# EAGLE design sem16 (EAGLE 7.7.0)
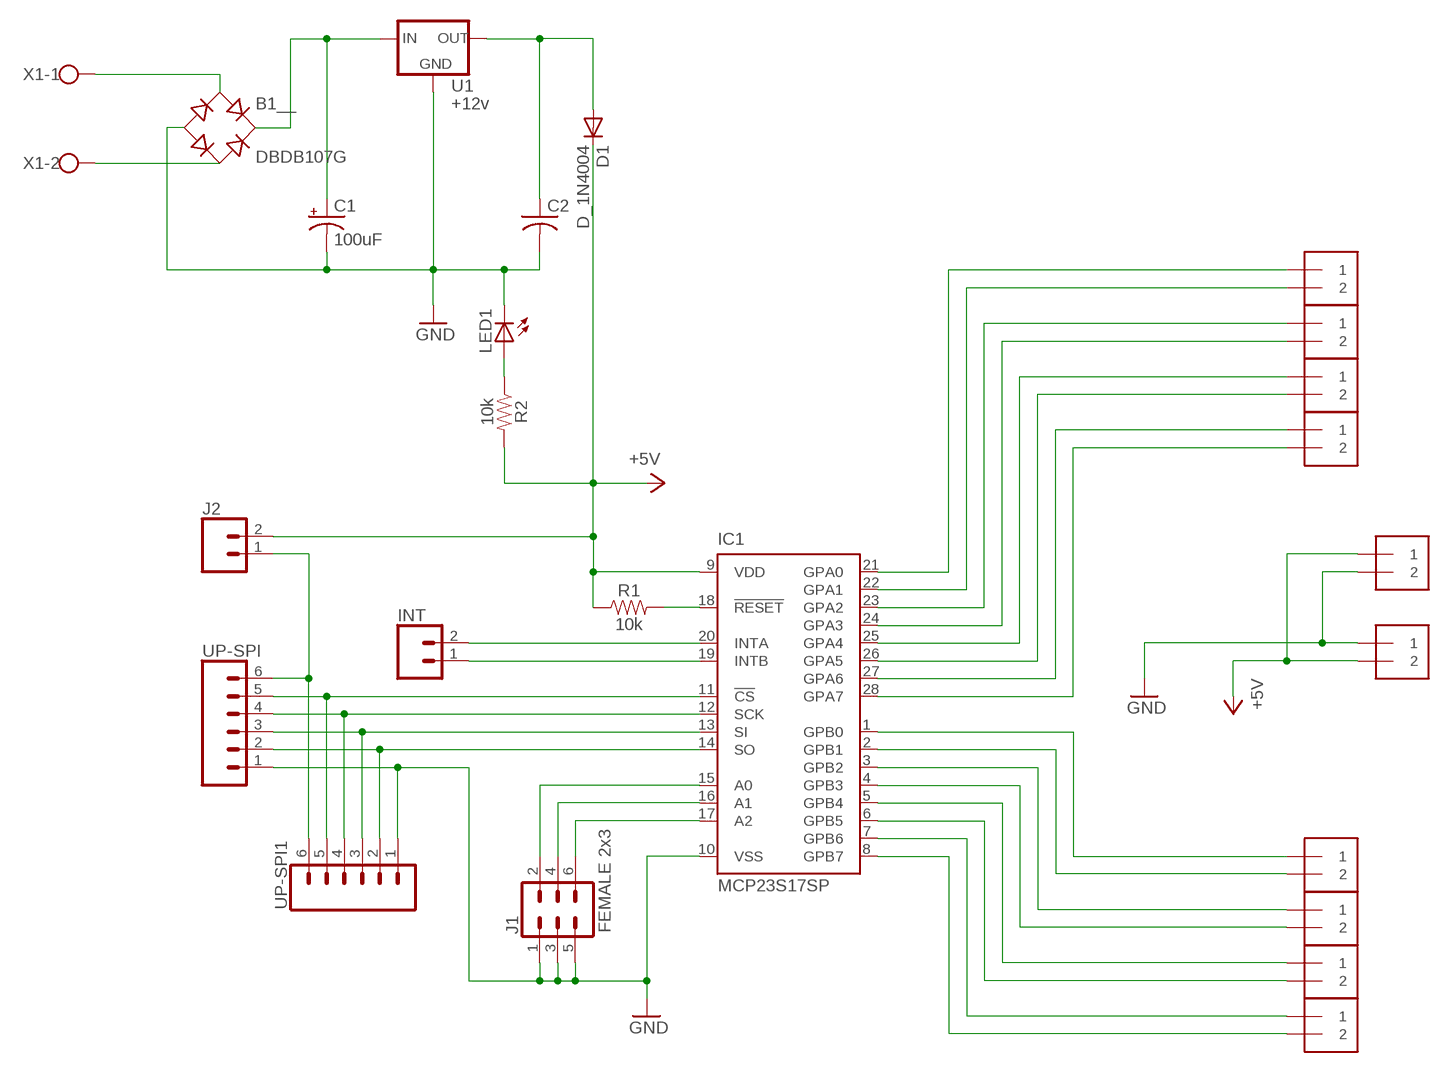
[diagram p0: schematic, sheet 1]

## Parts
+5V  1X2-3.5MM  [1X2-3.5MM]
A0_A1  1X2-3.5MM  [1X2-3.5MM]
A2_A3  1X2-3.5MM  [1X2-3.5MM]
A4_A5  1X2-3.5MM  [1X2-3.5MM]
A6_A7  1X2-3.5MM  [1X2-3.5MM]
B0_B1  1X2-3.5MM  [1X2-3.5MM]
B1__  DBDB107G  [DB]
B2_B3  1X2-3.5MM  [1X2-3.5MM]
B4_B5  1X2-3.5MM  [1X2-3.5MM]
B6_B7  1X2-3.5MM  [1X2-3.5MM]
C1  100uF  100UF-POLAR-RADIAL-2.5MM-25V-20%  [CPOL-RADIAL-2.5MM-6.5MM]
C2  C-US025-025X050  [C025-025X050]
D1  D_1N4004  [DO41-10]
GND  1X2-3.5MM  [1X2-3.5MM]
IC1  MCP23S17SP  [DIL28-3]
INT  CONN_02  [1X02]
J1  FEMALE 2x3  CONN_03X2FEMALE  [2X3]
J2  CONN_02  [1X02]
LED1  LED3MM  [LED3MM]
R1  10k  10KOHM-HORIZ-1/4W-1%  [AXIAL-0.3]
R2  10k  10KOHM-HORIZ-1/4W-1%  [AXIAL-0.3]
U1  +12v  V_REG_78XX7812  [TO-252]
UP-SPI  CONN_06LONGPADS  [1X06_LONGPADS]
UP-SPI1  CONN_06LONGPADS  [1X06_LONGPADS]
X1  W237-102  [W237-102]

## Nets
+5V: +5V.2 D1.C GND.1 IC1.9(VDD) J2.2 R1.P$1 R2.P$2
GND: +5V.1 B1__.- C1.2(-) C2.2 GND.2 IC1.10(VSS) J1.1 J1.3 J1.5 LED1.K(C) U1.3(GND) UP-SPI1.1 UP-SPI.1
N$1: IC1.11(!CS) UP-SPI1.5 UP-SPI.5
N$2: A0_A1.1 IC1.21(GPA0)
N$3: A0_A1.2 IC1.22(GPA1)
N$4: A2_A3.1 IC1.23(GPA2)
N$5: A2_A3.2 IC1.24(GPA3)
N$6: A4_A5.1 IC1.25(GPA4)
N$7: A4_A5.2 IC1.26(GPA5)
N$8: A6_A7.1 IC1.27(GPA6)
N$9: A6_A7.2 IC1.28(GPA7)
N$10: B0_B1.1 IC1.1(GPB0)
N$11: B0_B1.2 IC1.2(GPB1)
N$12: B2_B3.1 IC1.3(GPB2)
N$13: B2_B3.2 IC1.4(GPB3)
N$14: B4_B5.1 IC1.5(GPB4)
N$15: B4_B5.2 IC1.6(GPB5)
N$16: B6_B7.1 IC1.7(GPB6)
N$17: B6_B7.2 IC1.8(GPB7)
N$18: IC1.12(SCK) UP-SPI1.4 UP-SPI.4
N$19: IC1.13(SI) UP-SPI1.3 UP-SPI.3
N$20: IC1.14(SO) UP-SPI1.2 UP-SPI.2
N$22: B1__.+ C1.1(+) U1.1(IN)
N$23: IC1.19(INTB) INT.1
N$24: IC1.17(A2) J1.6
N$25: IC1.16(A1) J1.4
N$26: IC1.15(A0) J1.2
N$27: IC1.20(INTA) INT.2
N$28: IC1.18(!RESET) R1.P$2
N$30: C2.1 D1.A U1.2(OUT)
N$49: J2.1 UP-SPI1.6 UP-SPI.6
N$50: LED1.A R2.P$1
N$51: B1__.AC1 X1.1
N$52: B1__.AC2 X1.2

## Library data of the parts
+5V A0_A1 A2_A3 A4_A5 A6_A7 B0_B1 B2_B3 B4_B5 B6_B7 GND = servorail_v3:1X2: 3.5mm Terminal block
B1__ = rectifier:DB?*G: Single Phase 1.0 AMP Glass Passivated Bridge Rectifier Taiwan Semiconductor Co.,Ltd. - TSC Source: http://www.taiwansemi.com/TSCbig5/ezcatfiles/cust/img/img/db101g.pdf http://www.ts.com.tw/db/pictures/modules/PDT/PDT060207001/DBLS201G.pdf
C1 = SparkFun-Capacitors:100UF-POLAR: 100µF polarized capacitors; PROD_ID: CAP-08439
C2 = adafruit:C-US: CAPACITOR, American symbol
D1 = plg-rms:D_1N4004: DIODE
IC1 = plg-rms:MCP23S17: http://ww1.microchip.com/downloads/en/DeviceDoc/21952a.pdf Source: http://ww1.microchip.com/downloads/en/DeviceDoc/21952a.pdf; MF: MICROCHIP; MPN: MCP23S17-E/SP; OC_FARNELL: 1292238; OC_NEWARK: 31K2951
INT = SparkFun-Connectors:CONN_02: Multi connection point. Often used as Generic Header-pin footprint for 0.1 inch spaced/style header connections
J1 = SparkFun-Connectors:CONN_03X2: Multi connection point. Often used as Generic Header-pin footprint for 0.1 inch spaced/style header connections You can populate with any combo of single row headers, but if you'd like an exact match, check these: Header - 2x3 (Male, 0.1") (PRT-12807) Header - 2x3 (Female, 0.1") (PRT-13010) 2x3 Pin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; PROD_ID: CONN-11566
J2 = plg-rms:CONN_02: Multi connection point. Often used as Generic Header-pin footprint for 0.1 inch spaced/style header connections
LED1 = plg-rms:LED: LED
R1 R2 = SparkFun-Resistors:10KOHM: 10kΩ resistor; PROD_ID: RES-12183
U1 = SparkFun-IC-Power:V_REG_78XX: Voltage Regulator Standard 78xx regulator. IGO (Input Ground Output). Spark Fun Electronics SKU : COM-00107; PROD_ID: VREG-12370
UP-SPI UP-SPI1 = SparkFun-Connectors:CONN_06: Multi connection point. Often used as Generic Header-pin footprint for 0.1 inch spaced/style header connections On any of the 0.1 inch spaced packages, you can populate with these: Break Away Headers - Straight (PRT-00116) Break Away Male Headers - Right Angle (PRT-00553) Female Headers (PRT-00115)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
X1 = plg-rms:W237-102: WAGO SCREW CLAMP; MPN: 237-102; OC_FARNELL: unknown; OC_NEWARK: 70K9898

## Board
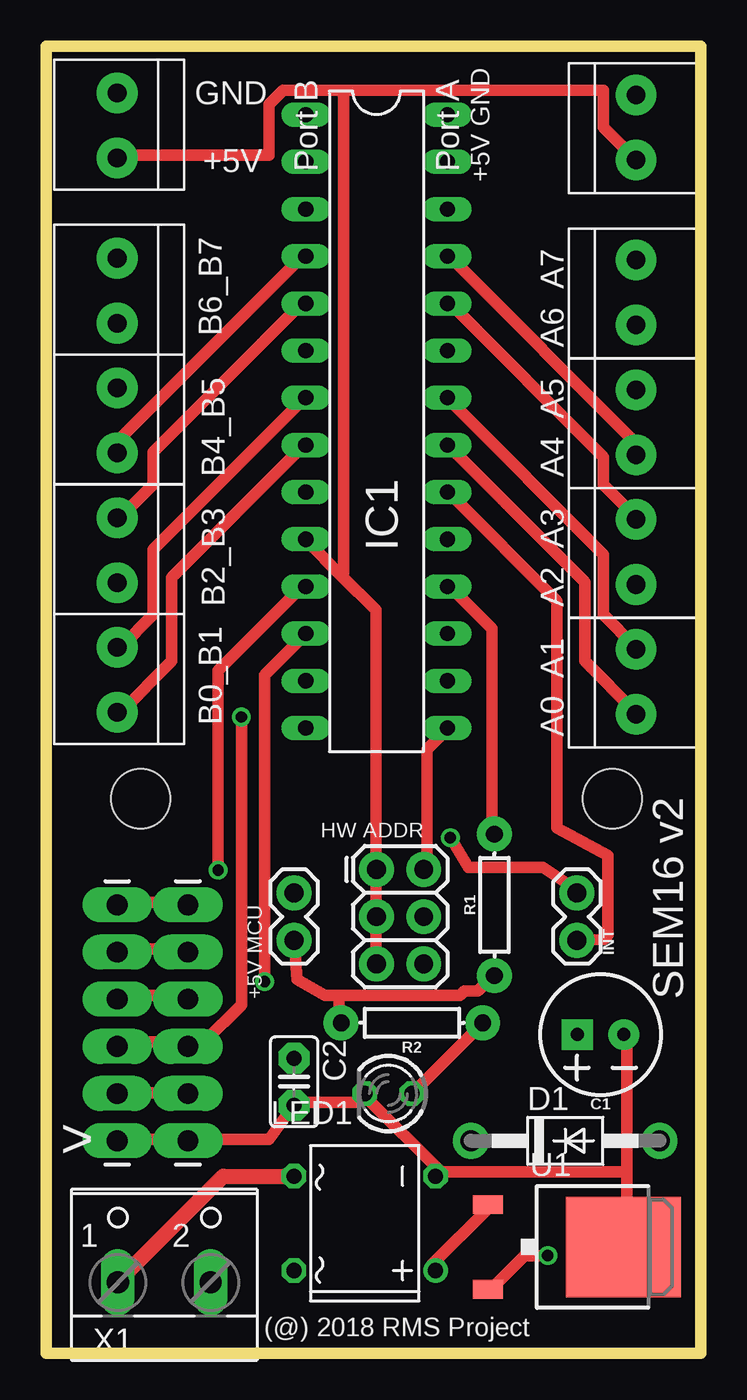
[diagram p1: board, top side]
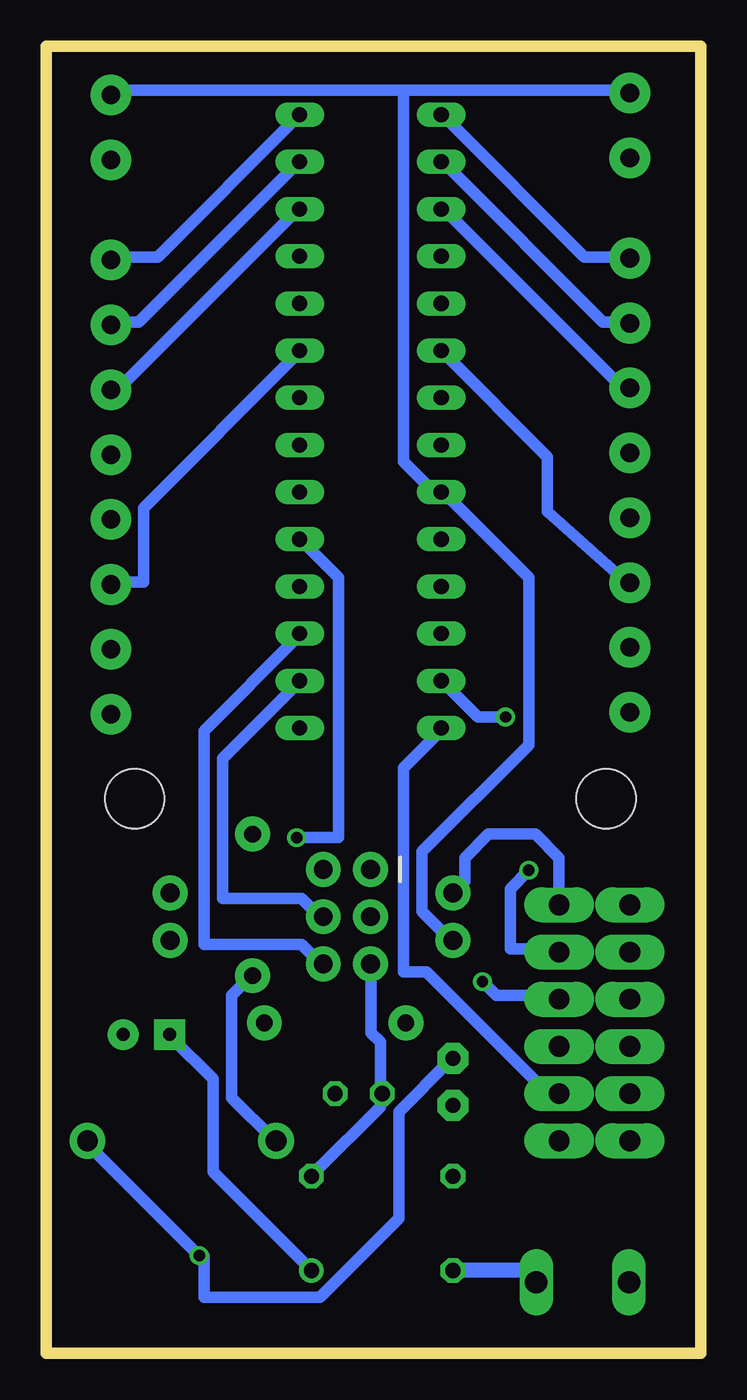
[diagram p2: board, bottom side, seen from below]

Size 35.23 x 70.35 mm. Coordinates in mm from the lower left corner, seen from the top.
Outline: 0,0 35.23,0 35.23,70.35 0,70.35 0,0
Copper layers (1*16): Top 0.035mm / dielectric 1.5mm / Bottom 0.035mm
Design rules "default *": minimum track width 24mil, minimum drill 24mil, track to track 12mil, track to pad 12mil, pad to pad 12mil, via to via 12mil, smd to smd 8mil, copper to edge 40mil, drill to drill 8mil, minimum pad ring 10mil, minimum via ring 8mil, stop-mask expansion 4mil, vias tented up to drill 0mil, thermal gap 10mil
Holes 3.2 mm at 5.08,29.84 30.48,29.84

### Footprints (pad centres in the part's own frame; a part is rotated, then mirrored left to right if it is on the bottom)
1X2-3.5MM = drill 1 pad 2.184: 1 1.8,0; 2 -1.7,0
DB = drill 0.813: + -2.54,-3.81 | drill 0.813 octagon: - 2.54,-3.81; AC1 2.54,3.81; AC2 -2.54,3.81
CPOL-RADIAL-2.5MM-6.5MM = drill 0.7 pad 1.651 square: 1 1.25,0 | drill 0.7 pad 1.651: 2 -1.25,0
C025-025X050 = drill 0.813 pad 1.676 octagon: 1 -1.27,0; 2 1.27,0
DO41-10 = drill 1.118 pad 1.93: A 5.08,0; C -5.08,0
DIL28-3 = drill 0.813 long: 1 -16.51,-3.81; 2 -13.97,-3.81; 3 -11.43,-3.81; 4 -8.89,-3.81; 5 -6.35,-3.81; 6 -3.81,-3.81; 7 -1.27,-3.81; 8 1.27,-3.81; 9 3.81,-3.81; 10 6.35,-3.81; 11 8.89,-3.81; 12 11.43,-3.81; 13 13.97,-3.81; 14 16.51,-3.81; 15 16.51,3.81; 16 13.97,3.81; 17 11.43,3.81; 18 8.89,3.81; 19 6.35,3.81; 20 3.81,3.81; 21 1.27,3.81; 22 -1.27,3.81; 23 -3.81,3.81; 24 -6.35,3.81; 25 -8.89,3.81; 26 -11.43,3.81; 27 -13.97,3.81; 28 -16.51,3.81
1X02 = drill 1.016 pad 1.88: 1 0,0; 2 2.54,0
2X3 = drill 1.016 pad 1.88: 1 0,0; 2 0,2.54; 3 2.54,0; 4 2.54,2.54; 5 5.08,0; 6 5.08,2.54
LED3MM = drill 0.813 octagon: A -1.27,0; K 1.27,0
AXIAL-0.3 = drill 0.9 pad 1.88: P$1 -3.81,0; P$2 3.81,0
TO-252 = smd 1 x 1.6: 1 -2.28,-4.8; 2 2.28,-4.8 | smd 5.4 x 6.2: 3 0,2.5
1X06_LONGPADS = drill 1.118 pad 1.88 long: 1 0,0; 2 2.54,0; 3 5.08,0; 4 7.62,0; 5 10.16,0; 6 12.7,0
W237-102 = drill 1.194 long: 1 -2.5,-1.27; 2 2.5,-1.27

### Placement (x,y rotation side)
+5V  31.75,66.04 270 top
A0_A1  31.75,36.2 270 top
A2_A3  31.75,43.18 270 top
A4_A5  31.75,50.16 270 top
A6_A7  31.75,57.15 270 top
B0_B1  3.81,57.15 90 top
B1__  17.14,6.99 90 top
B2_B3  3.81,50.16 90 top
B4_B5  3.81,43.18 90 top
B6_B7  3.81,36.2 90 top
C1  29.84,17.14 180 top
C2  13.34,14.61 270 top
D1  27.94,11.43 0 top
GND  3.81,66.04 90 top
IC1  17.78,50.16 270 top
INT  28.57,24.77 270 top
J1  17.78,26.04 270 top
J2  13.34,24.77 270 top
LED1  18.41,13.97 180 top
R1  24.13,24.13 90 top
R2  19.68,17.78 180 top
U1  28.57,5.71 270 top
UP-SPI  7.62,11.43 90 top
UP-SPI1  3.81,11.43 90 top
X1  6.35,5.08 0 top

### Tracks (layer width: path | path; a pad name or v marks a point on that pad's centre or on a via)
+5V
  Top 0.61: 15.75,19.25 15.75,18 R2.P$2 | J2.2 13.5,20.11 15,19.25 15.75,19.25 | 15.75,19.25 22.27,19.25 22.52,19.5 23.25,19.5 24,20.25 R1.P$1
  Bottom 0.61: 16,68 31.75,68 +5V.2 | 16,68 4,68 GND.1 | J2.2 13.5,22.27 15,23.77 15,27 9.25,32.75 9.25,41.75 13.75,46.25 IC1.9 14.25,46.25 16,48 16,68 | D1.C 23,11.5 25.25,13.75 25.25,19.25 24.25,20.25 R1.P$1
GND
  Top 0.61: 16,68 30,68 30,66 +5V.1 | 16,68 12.75,68 12,67.25 12,64.5 4,64.5 GND.2 | 15.88,41.88 17.75,40 17.75,26.25 J1.1 17.75,25.75 17.75,23.75 J1.3 17.75,23.25 17.75,21.25 J1.5 | 15.88,41.88 14,43.75 IC1.10 | UP-SPI1.1 4,11.5 7.5,11.5 UP-SPI.1 7.75,11.5 11.98,11.5 13.25,13.25 C2.2 13.5,13.5 16.75,13.5 17,13.75 LED1.K 17.25,13.75 21.25,9.75 31.25,9.75 | 16,68 16,42 15.88,41.88 | 31.25,9.75 31.25,5.75 U1.3 | 31.25,9.75 31.25,17 C1.2
  Bottom 0.61: J1.5 17.75,20.75 17.75,17.25 17.25,16.75 17.25,14.25 LED1.K 17.25,13.75 17.25,13.25 20.75,9.75 B1__.-
N$1  (via drill 0.61)
  Top 0.61: v9.25,26 9.25,36.75 13.75,41.25 IC1.11 | UP-SPI1.5 4,21.75 7.5,21.75 UP-SPI.5
  Bottom 0.61: v9.25,26 10.25,25 10.25,21.75 7.75,21.75 UP-SPI.5
N$2
  Top 0.61: IC1.21 21.75,48.75 29,41.5 29,37.25 31.75,34.5 A0_A1.1
N$3
  Top 0.61: IC1.22 21.75,51.25 30,43 30,39.75 31.75,38 A0_A1.2
N$4
  Bottom 0.61: IC1.23 21.75,53.75 30,45.5 30,41.5 31.75,41.5 A2_A3.1
N$5
  Top 0.61: IC1.24 21.75,56.5 30,48.25 30,46.75 31.75,45 A2_A3.2
N$6
  Top 0.61: A4_A5.1 31.75,49 21.75,59 IC1.25
N$7
  Bottom 0.61: IC1.26 21.75,61.5 31.25,52 31.75,52 A4_A5.2
N$8
  Bottom 0.61: IC1.27 21.75,64 30.25,55.5 31.75,55.5 A6_A7.1
N$9
  Bottom 0.61: IC1.28 21.75,66.5 29.25,59 31.75,59 A6_A7.2
N$10
  Bottom 0.61: IC1.1 13.75,66.5 6.25,59 4,59 B0_B1.1
N$11
  Bottom 0.61: IC1.2 13.75,64 5.25,55.5 4,55.5 B0_B1.2
N$12
  Bottom 0.61: IC1.3 13.75,61.5 4.25,52 4,52 B2_B3.1
N$13
  Top 0.61: IC1.4 13.75,59 4,49.25 4,48.5 B2_B3.2
N$14
  Top 0.61: IC1.5 13.75,56.5 5.75,48.5 5.75,46.75 4,45 B4_B5.1
N$15
  Bottom 0.61: IC1.6 13.75,53.75 8.25,48.25 8.25,45.31 4,41.5 B4_B5.2
N$16
  Top 0.61: IC1.7 13.75,51.25 5.75,43.25 5.75,39.75 4,38 B6_B7.1
N$17
  Top 0.61: IC1.8 13.75,48.75 6.75,41.75 6.75,37.25 4,34.5 B6_B7.2
N$18  (via drill 0.61)
  Top 0.61: v11.75,20 11.75,36.5 13.75,38.5 IC1.12 | UP-SPI1.4 4,19.25 7.5,19.25 UP-SPI.4
  Bottom 0.61: v11.75,20 11,19.25 7.75,19.25 UP-SPI.4
N$19  (via drill 0.61)
  Top 0.61: v10.5,34.25 10.5,18.75 8.5,16.75 7.75,16.75 UP-SPI.3 7.5,16.75 4,16.75 UP-SPI1.3
  Bottom 0.61: v10.5,34.25 12,34.25 13.75,36 IC1.13
N$20
  Top 0.61: UP-SPI1.2 4,14 7.5,14 UP-SPI.2
  Bottom 0.61: IC1.14 14,33.5 16,31.5 16,20.52 14.77,20.52 8.25,14 7.75,14 UP-SPI.2
N$22
  Top 0.61: U1.1 23.75,7.75 20.75,4.75 20.75,4.5 B1__.+
  Bottom 0.61: C1.1 28.5,17 26.25,14.75 26.25,9.75 21,4.5 B1__.+
N$23  (via drill 0.61)
  Top 0.61: v21.75,27.75 22.73,26.14 26.73,26.14 28.5,25 INT.1
  Bottom 0.61: v21.75,27.75 19.5,27.75 19.5,41.75 21.5,43.75 IC1.19
N$24
  Bottom 0.61: IC1.17 21.75,38.5 26.75,33.5 26.75,22 21.5,22 20.5,21 J1.6
N$25
  Bottom 0.61: IC1.16 21.75,36 25.75,32 25.75,24.48 21.48,24.48 20.5,23.5 J1.4
N$26
  Top 0.61: IC1.15 21.5,33.5 20.5,32.5 20.5,26.25 J1.2
N$27
  Top 0.61: IC1.20 21.75,46.25 27.5,40.5 27.5,28.27 30.25,26.79 30.25,22.5 30.02,22.27 INT.2
N$28
  Top 0.61: IC1.18 21.75,41.25 24,39 24,28 R1.P$2
N$30  (via drill 0.61)
  Top 0.61: v27,5.25 25.75,5.25 24,3.5 U1.2
  Bottom 0.61: D1.A 33,11.25 v27,5.25 26.75,5.25 26.75,3 20.5,3 16.25,7.25 16.25,13 13.5,15.75 C2.1
N$49
  Top 0.61: UP-SPI1.6 4,24.25 7.5,24.25 UP-SPI.6
  Bottom 0.61: J2.1 12.7,25.4 12.7,26.67 11.43,27.94 8.89,27.94 7.62,26.67 UP-SPI.6
N$50
  Top 0.61: LED1.A 19.75,14 23.25,17.5 23.25,17.75 R2.P$1
N$51
  Top 0.61: 13.25,9.5 B1__.AC1 | 4,4 X1.1
  Top 0.813: 4,4 9.53,9.53 B1__.AC1
N$52
  Bottom 0.813: X1.2 9.48,4.45 B1__.AC2

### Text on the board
tNames: Port B | Port A | +5V GND | HW ADDR | +5V MCU | SEM16 v2 | > | (@) 2018 RMS Project

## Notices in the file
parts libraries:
SparkFun-IC-Power: Licensing: Creative Commons ShareAlike 4.0 International - https://creativecommons.org/licenses/by-sa/4.0
